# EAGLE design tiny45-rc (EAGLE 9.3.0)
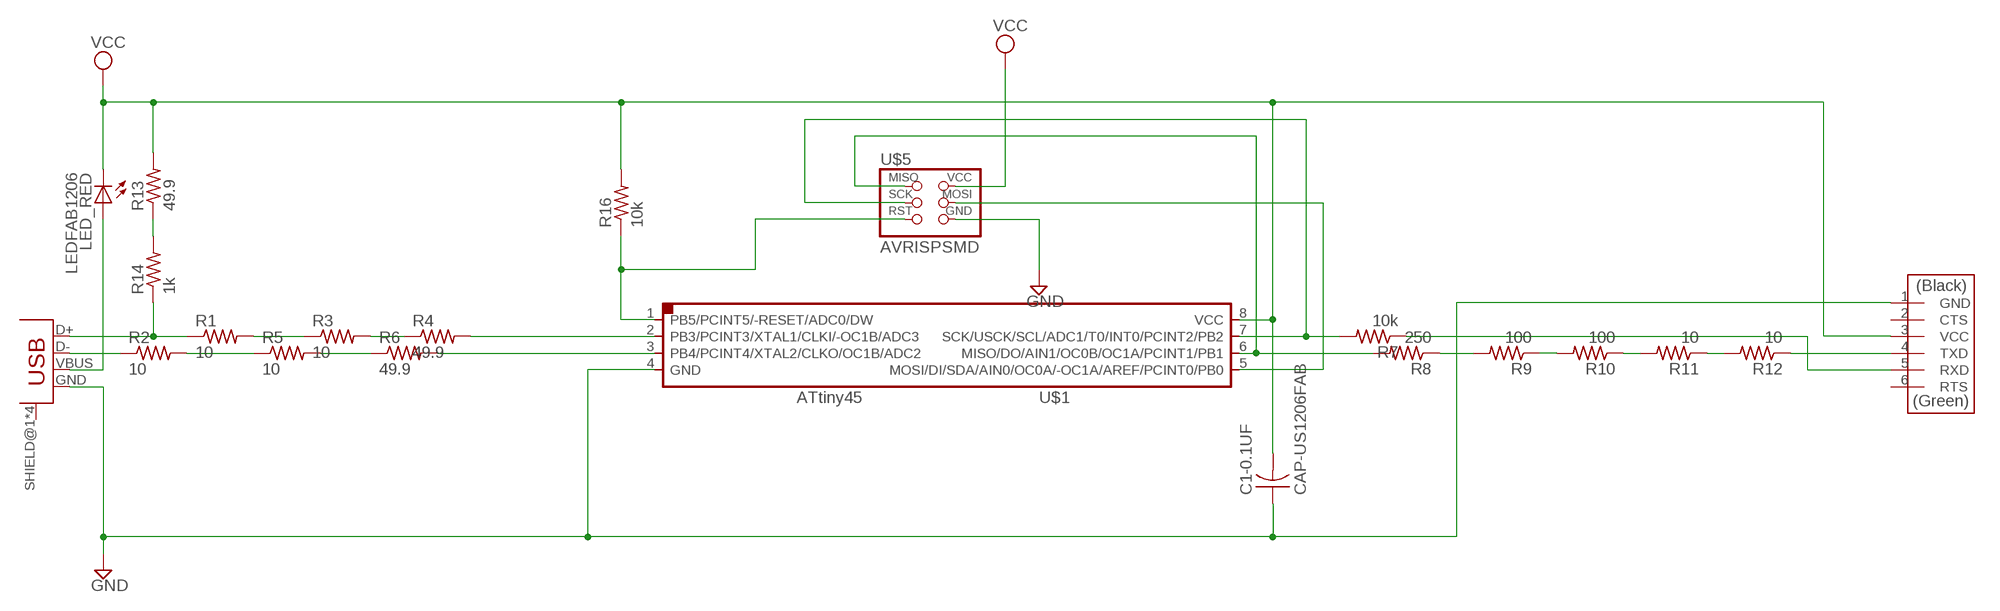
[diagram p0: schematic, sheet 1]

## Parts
C1-0.1UF  CAP-US1206FAB  [C1206FAB]
LED_RED  LEDFAB1206  [LED1206FAB]
R1  10  RES-US1206FAB  [R1206FAB]
R2  10  RES-US1206FAB  [R1206FAB]
R3  10  RES-US1206FAB  [R1206FAB]
R4  49.9  RES-US1206FAB  [R1206FAB]
R5  10  RES-US1206FAB  [R1206FAB]
R6  49.9  RES-US1206FAB  [R1206FAB]
R7  10k  RES-US1206FAB  [R1206FAB]
R8  250  RES-US1206FAB  [R1206FAB]
R9  100  RES-US1206FAB  [R1206FAB]
R10  100  RES-US1206FAB  [R1206FAB]
R11  10  RES-US1206FAB  [R1206FAB]
R12  10  RES-US1206FAB  [R1206FAB]
R13  49.9  RES-US1206FAB  [R1206FAB]
R14  1k  RES-US1206FAB  [R1206FAB]
R16  10k  RES-US1206FAB  [R1206FAB]
U$1  ATTINY45SI  [SOIC8]
U$2  USB_MINIB  [USB_MINIB]
U$3  FTDI-SMD-HEADER  [1X06SMD]
U$5  AVRISPSMD  [2X03SMD]

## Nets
GND: C1-0.1UF.1 U$1.4(GND) U$2.GND U$3.1(GND) U$5.6(GND)
N$1: R1.1 R14.1 U$2.D+
N$2: R4.2 U$1.2(PB3/PCINT3/XTAL1/CLKI/-OC1B/ADC3)
N$3: R2.2 R5.1
N$4: R2.1 U$2.D-
N$5: R5.2 R6.1
N$6: R6.2 U$1.3(PB4/PCINT4/XTAL2/CLKO/OC1B/ADC2)
N$7: R1.2 R3.1
N$8: R3.2 R4.1
N$9: R7.2 U$1.7(SCK/USCK/SCL/ADC1/T0/INT0/PCINT2/PB2) U$5.3(SCK)
N$10: R8.2 U$1.6(MISO/DO/AIN1/OC0B/OC1A/PCINT1/PB1) U$5.1(MISO)
N$11: R8.1 R9.2
N$12: R9.1 R10.2
N$13: R10.1 R11.2
N$14: R11.1 R12.2
N$15: R12.1 U$3.4(TXD)
N$16: R7.1 U$3.5(RXD)
N$17: R13.1 R14.2
N$18: LED_RED.1(A) U$2.VBUS
N$20: R16.1 U$1.1(PB5/PCINT5/-RESET/ADC0/DW) U$5.5(RST)
N$24: U$1.5(MOSI/DI/SDA/AIN0/OC0A/-OC1A/AREF/PCINT0/PB0) U$5.4(MOSI)
VCC: C1-0.1UF.2 LED_RED.2(C) R13.2 R16.2 U$1.8(VCC) U$3.3(VCC) U$5.2(VCC)
Unconnected: U$2.SHIELD@1(SHIELD) U$2.SHIELD@2(SHIELD) U$2.SHIELD@3(SHIELD) U$2.SHIELD@4(SHIELD) U$3.2(CTS) U$3.6(RTS)

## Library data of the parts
C1-0.1UF = fab:CAP-US
LED_RED = fab:LED: LED
R1-R14 R16 = fab:RES-US: Resistor (US Symbol)
U$1 = fab:ATTINY45
U$2 = fab:USB_MINIB
U$3 = fab:FTDI-SMD-HEADER
U$5 = fab:AVRISP

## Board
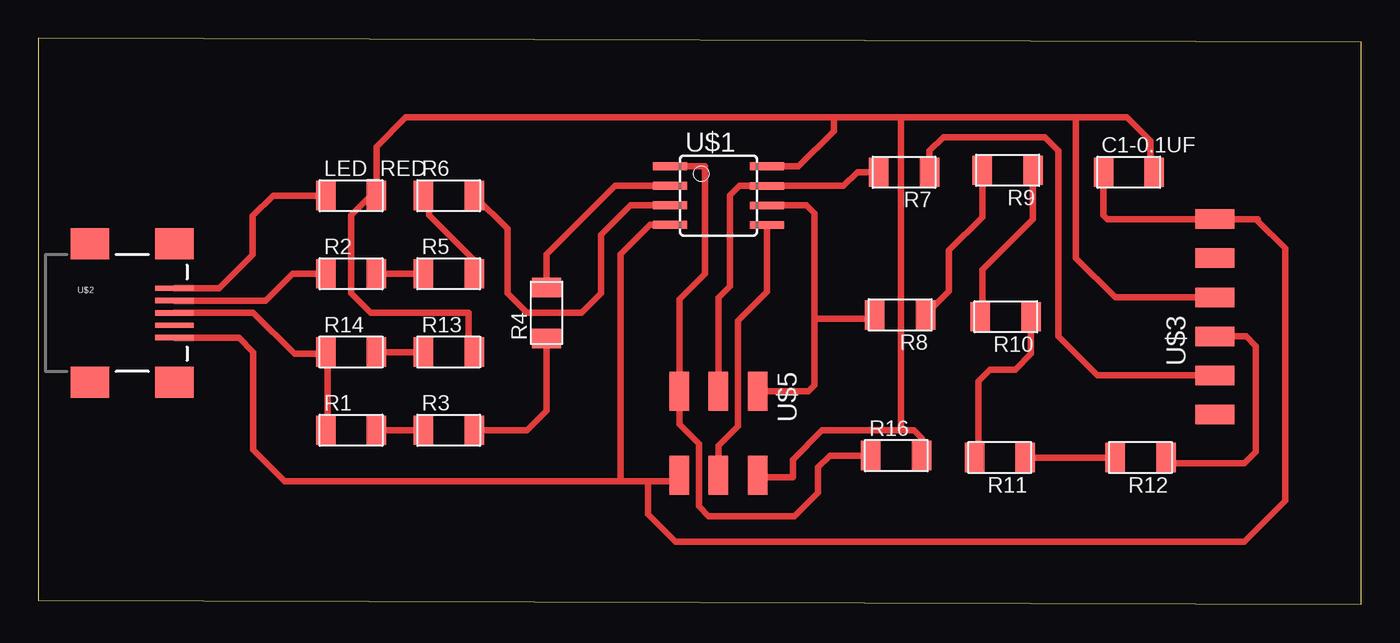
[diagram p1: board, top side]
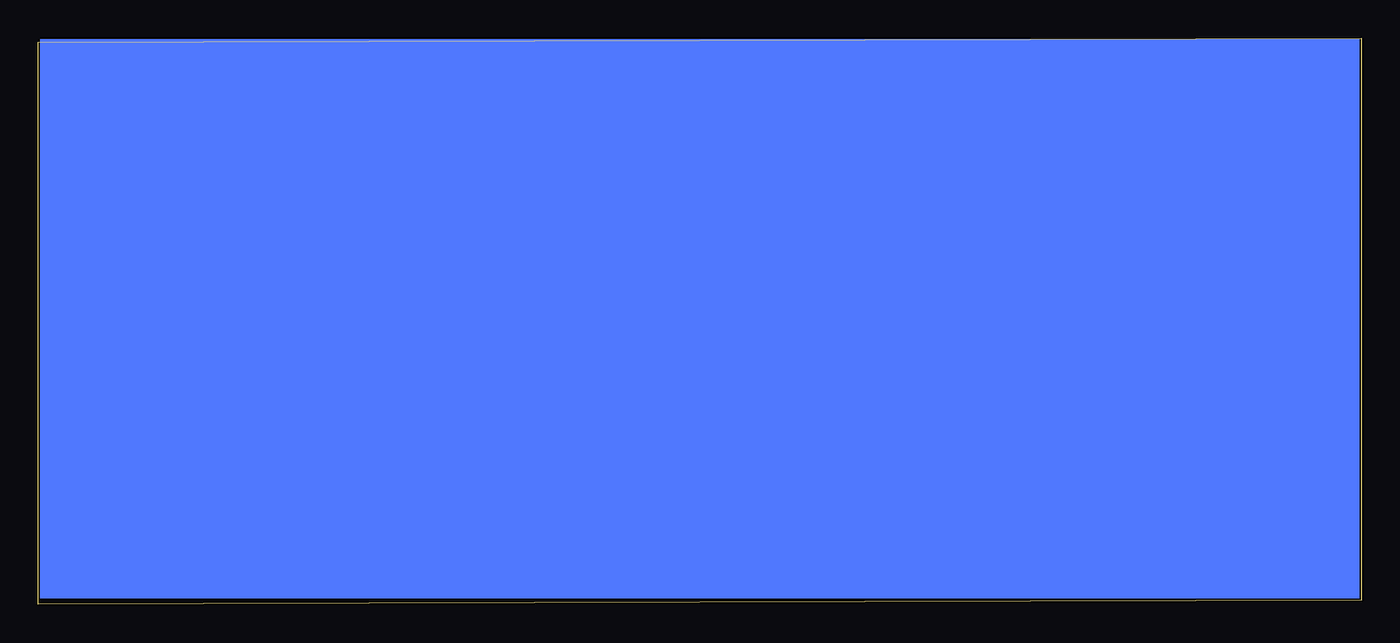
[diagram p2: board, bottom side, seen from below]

Size 85.96 x 36.75 mm. Coordinates in mm from the lower left corner, seen from the top.
Outline: 0,0.25 85.96,0 85.96,36.5 0,36.75 0,0.25
Copper layers (1*16): Top 0.035mm / dielectric 1.5mm / Bottom 0.035mm
Design rules "default": minimum track width 6mil, minimum drill 0.35mm, track to track 6mil, track to pad 6mil, pad to pad 6mil, via to via 6mil, smd to smd 6mil, copper to edge 40mil, drill to drill 6mil, minimum pad ring 10mil, minimum via ring 8mil, stop-mask expansion 4mil, vias tented up to drill 0mil, thermal gap 10mil

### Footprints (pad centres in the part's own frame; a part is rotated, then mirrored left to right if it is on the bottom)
C1206FAB = smd 1.27 x 1.905: 1 -1.651,0; 2 1.651,0
LED1206FAB = smd 1.27 x 1.905: 1 -1.651,0; 2 1.651,0
R1206FAB = smd 1.27 x 1.905: 1 -1.651,0; 2 1.651,0
SOIC8 = smd 0.5 x 2.2: 1 -1.905,-3.154; 2 -0.645,-3.154; 3 0.625,-3.154; 4 1.895,-3.154; 5 1.905,3.154; 6 0.635,3.154; 7 -0.635,3.154; 8 -1.905,3.154
USB_MINIB = smd 2.5 x 0.35: D+ 3.77,0; D- 3.77,0.8; GND 3.77,-1.6; ID 3.77,-0.8; VBUS 3.77,1.6 | smd 2.5 x 2: SHIELD@1 -1.73,-4.5; SHIELD@2 -1.73,4.5; SHIELD@3 3.77,4.5; SHIELD@4 3.77,-4.5
1X06SMD = smd 2.54 x 1.27: 1 0,6.35; 2 0,3.81; 3 0,1.27; 4 0,-1.27; 5 0,-3.81; 6 0,-6.35
2X03SMD = smd 2.54 x 1.27: 1 -2.54,2.54; 2 2.92,2.54; 3 -2.54,0; 4 2.92,0; 5 -2.54,-2.54; 6 2.92,-2.54

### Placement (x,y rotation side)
C1-0.1UF  70.87,28.07 0 top
LED_RED  20.32,26.54 0 top
R1  20.32,11.3 0 top
R2  20.32,21.46 0 top
R3  26.67,11.3 0 top
R4  33.02,18.92 90 top
R5  26.67,21.46 0 top
R6  26.67,26.54 0 top
R7  56.26,28.07 180 top
R8  56.01,18.8 180 top
R9  62.99,28.19 180 top
R10  62.87,18.67 180 top
R11  62.48,9.53 180 top
R12  71.63,9.53 180 top
R13  26.67,16.38 0 top
R14  20.32,16.38 0 top
R16  55.75,9.65 0 top
U$1  44.2,26.54 270 top
U$2  5.08,18.92 0 top
U$3  76.45,18.67 0 top
U$5  44.2,11.3 270 top

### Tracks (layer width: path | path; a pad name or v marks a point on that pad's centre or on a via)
GND
  Top 0.152: 41.81,8 U$5.6 | 41.15,24.66 U$1.4
  Top 0.406: U$2.GND 13.03,17.32 13.97,16.38 13.97,10.03 16,8 37.85,8 | 37.85,8 39.62,8 | 39.62,8 41.81,8 | U$1.4 39.76,24.65 37.85,22.73 37.85,8 | C1-0.1UF.1 69.22,25.27 69.47,25.02 U$3.1 79.25,25.02 79.25,24.89 81.03,23.11 81.03,6.73 78.36,4.06 41.4,4.06 39.62,5.84 39.62,8
N$1
  Top 0.152: 18.8,11.4 R1.1 | 8.99,18.82 U$2.D+
  Top 0.406: U$2.D+ 13.97,18.92 16.64,16.26 18.8,16.26 | R14.1 18.8,16.26 | 18.8,16.26 18.8,11.4
N$2
  Top 0.152: 41,27.1 U$1.2
  Top 0.406: R4.2 33.02,22.73 37.47,27.19 U$1.2
N$3
  Top 0.406: R2.2 R5.1
N$4
  Top 0.152: 8.99,19.74 U$2.D-
  Top 0.406: U$2.D- 14.77,19.72 16.51,21.46 R2.1
N$5
  Top 0.406: R6.1 25.4,26.16 25.4,25.27 28.32,22.35 R5.2
N$6
  Top 0.152: R6.2 28.98,25.88 | 41,25.88 U$1.3
  Top 0.406: R6.2 30.48,24.38 30.48,20.19 31.75,18.92 35.31,18.92 36.58,20.19 36.58,24 38.48,25.91 | 38.49,25.92 38.48,25.91 | U$1.3 41.03,25.91 38.48,25.91
N$7
  Top 0.406: R1.2 R3.1
N$8
  Top 0.406: R3.2 31.75,11.3 33.02,12.57 R4.1
N$9
  Top 0.406: U$5.3 44.2,19.91 44.95,20.67 44.95,26.56 45.57,27.18 U$1.7 52.32,27.18 53.21,28.07 R7.2
N$10
  Top 0.152: 47.4,25.88 U$1.6
  Top 0.406: U$1.6 49.91,25.91 50.42,25.4 50.42,18.54 | 50.42,18.54 50.42,14.22 50.04,13.84 U$5.1 | R8.2 54.1,18.54 50.42,18.54
N$11
  Top 0.406: R8.1 59.18,20.32 59.18,22.99 61.34,25.15 R9.2
N$12
  Top 0.406: R10.2 61.34,18.8 61.34,21.72 64.64,25.02 R9.1
N$13
  Top 0.406: R11.2 61.09,9.78 61.09,14.48 61.85,15.24 63.5,15.24 64.52,16.26 R10.1
N$14
  Top 0.406: R11.1 R12.2
N$15
  Top 0.406: R12.1 73.66,9.14 78.36,9.14 79.12,9.91 79.12,16.76 78.49,17.4 U$3.4
N$16
  Top 0.152: U$3.5 76.4,14.86
  Top 0.406: R7.1 57.91,29.46 58.8,30.35 65.41,30.35 66.29,29.46 66.29,17.4 68.83,14.86 U$3.5
N$17
  Top 0.406: R14.2 R13.1
N$18
  Top 0.406: U$2.VBUS 11.76,20.52 13.93,22.69 13.93,25.23 15.24,26.54 LED_RED.1
N$20
  Top 0.152: 41.15,28.32 U$1.1
  Top 0.406: U$1.1 43.31,28.45 43.31,21.46 41.66,19.81 U$5.5 41.66,11.68 42.93,10.41 42.93,6.35 43.56,5.72 49.15,5.72 50.67,7.24 50.67,8.89 51.44,9.65 R16.1
N$24
  Top 0.406: U$1.5 47.35,20.3 45.47,18.41 45.47,11.56 44.2,10.29 U$5.4
VCC
  Top 0.152: 28.35,16.38 R13.2
  Top 0.406: R13.2 27.94,16.76 27.94,18.92 21.59,18.92 20.32,20.19 20.32,25.27 21.59,26.54 LED_RED.2 21.97,29.72 23.88,31.62 51.69,31.62 | U$5.2 46.86,8.26 49.02,8.26 49.02,9.4 50.93,11.3 56.01,11.3 | 56.01,11.3 56.9,11.3 57.4,10.79 R16.2 | 56.01,11.3 56.06,11.35 56.06,31.57 56.01,31.62 | U$1.8 49.4,28.45 51.69,30.73 51.69,31.62 | 51.69,31.62 56.01,31.62 | 56.01,31.62 67.44,31.62 | 67.44,31.62 70.74,31.62 72.26,30.1 72.26,28.32 C1-0.1UF.2 | 67.44,31.62 67.44,22.48 69.98,19.94 U$3.3
(copper drawn outside any net)
  shapes: Bottom area x1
